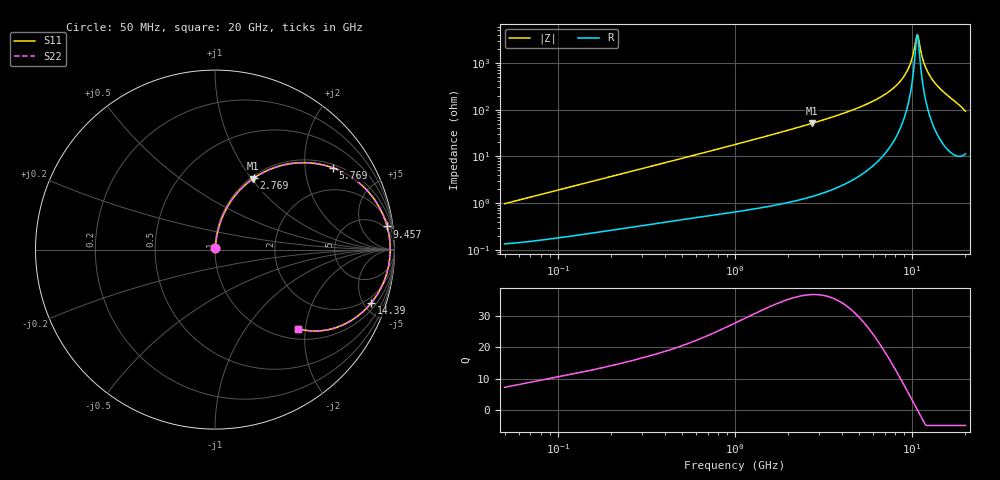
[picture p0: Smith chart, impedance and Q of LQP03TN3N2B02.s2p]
!Murata Part Number: LQP03TN3N2B02
!These Parameters are Measured in Series Mode Connection
!  o--[Z]--o
!Port1  Port2
!  o-------o
!Freq. Start=50[MHz] Stop=20[GHz], 401[Steps]
# Hz S RI R 50
!Freq.(Hz) S11(Real) S11(Imag) S21(Real) S21(Imag) S12(Real) S12(Imag) S22(Real) S22(Imag)
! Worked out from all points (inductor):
!   401 points, 50 MHz to 20 GHz, reference 50 ohm
!   read as one part in series: L = 3.05 nH near 51.52 MHz
!   highest Q = 36.9 at 2.728 GHz (marker M1), where L = 2.97 nH
!   self-resonance near 10.66 GHz
!   S11 on the Smith chart (normalised r, x): 50 MHz: 1.00, +0.02; 2.769 GHz: 1.03, +1.04; 5.769 GHz: 1.11, +2.81; 9.457 GHz: 3, +14; 14.39 GHz: 1.46, -5.61; 20 GHz: 1.23, -1.83
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5e7  0.00143 0.00959  0.9986 -0.00959  0.9986 -0.00959  0.00143 0.00959
1.364002e8  0.00276 0.0254  0.9972 -0.0254  0.9972 -0.0254  0.00276 0.0254
3.721004e8  0.0082 0.0667  0.9918 -0.0667  0.9918 -0.0667  0.0082 0.0667
1e9  0.0368 0.171  0.9632 -0.171  0.9632 -0.171  0.0368 0.171
1.766834e9  0.0992 0.2847  0.9008 -0.2847  0.9008 -0.2847  0.0992 0.2847
2.728004e9  0.2127 0.3959  0.7873 -0.3959  0.7873 -0.3959  0.2127 0.3959
2.769174e9  0.2182 0.3997  0.7818 -0.3997  0.7818 -0.3997  0.2182 0.3997
4.275624e9  0.4404 0.4816  0.5596 -0.4816  0.5596 -0.4816  0.4404 0.4816
5.769027e9  0.6576 0.4554  0.3424 -0.4554  0.3424 -0.4554  0.6576 0.4554
7.442007e9  0.8437 0.3336  0.1563 -0.3336  0.1563 -0.3336  0.8437 0.3336
8.516016e9  0.92 0.2276  0.08 -0.2276  0.08 -0.2276  0.92 0.2276
9.457416e9  0.9592 0.1288  0.0408 -0.1288  0.0408 -0.1288  0.9592 0.1288
9.892087e9  0.9694 0.0832  0.0306 -0.0832  0.0306 -0.0832  0.9694 0.0832
1.050288e10  0.976 0.0204  0.024 -0.0204  0.024 -0.0204  0.976 0.0204
1.082228e10  0.9762 -0.0115  0.0238 0.0115  0.0238 0.0115  0.9762 -0.0115
1.098561e10  0.9755 -0.0275  0.0245 0.0275  0.0245 0.0275  0.9755 -0.0275
1.166392e10  0.9672 -0.0915  0.0328 0.0915  0.0328 0.0915  0.9672 -0.0915
1.220001e10  0.9552 -0.1389  0.0448 0.1389  0.0448 0.1389  0.9552 -0.1389
1.314879e10  0.9242 -0.2151  0.0758 0.2151  0.0758 0.2151  0.9242 -0.2151
1.438523e10  0.8689 -0.2992  0.1311 0.2992  0.1311 0.2992  0.8689 -0.2992
1.747767e10  0.6788 -0.433  0.3212 0.433  0.3212 0.433  0.6788 -0.433
2e10  0.4645 -0.4408  0.5355 0.4408  0.5355 0.4408  0.4645 -0.4408
